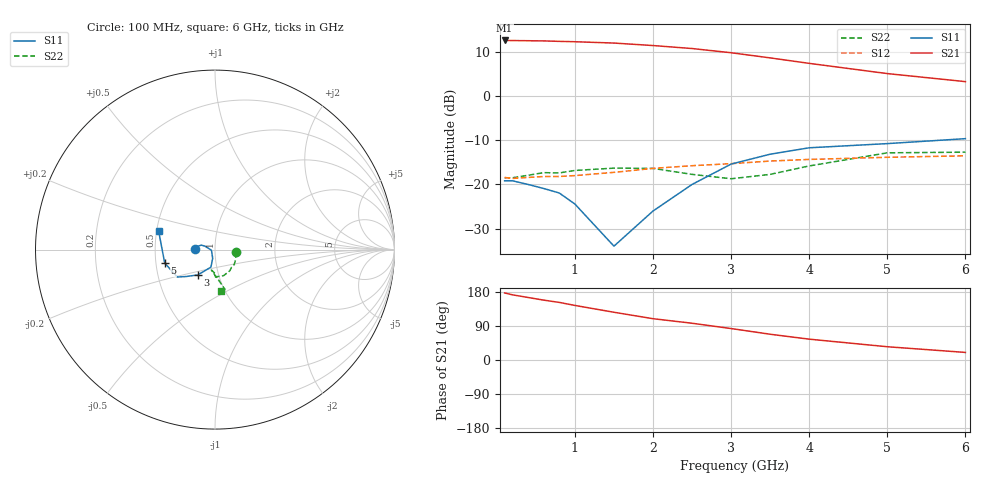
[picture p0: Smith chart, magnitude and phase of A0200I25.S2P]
!  MSA-0200 S AND NOISE PARAMETERS
!  Id=25mA  LAST UPDATED 07-22-92
# ghz s ma r 50
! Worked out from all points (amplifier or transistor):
!   14 points, 100 MHz to 6 GHz, reference 50 ohm
!   highest |S21| = 12.6 dB at 100 MHz (marker M1)
!   |S21| within 3 dB of that: start of sweep to 3.094 GHz
!   unconditionally stable (mu >= 1): start of sweep to end of sweep
!   at 400 MHz: K = 1.20, MAG = 12.8 dB, |S12| = -18.4 dB
!   at 2 GHz: K = 1.14, MAG = 11.7 dB, |S12| = -16.4 dB
!   at 6 GHz: K = 1.47, MAG = 4.3 dB, |S12| = -13.5 dB
!   lowest NFmin = 6.00 dB at 100 MHz
!   S11 on the Smith chart (normalised r, x): 100 MHz: 0.80, +0.00; 3 GHz: 0.80, -0.23; 5 GHz: 0.56, -0.09; 6 GHz: 0.51, +0.12
0.1  0.11 179.0  4.27 177.0  0.12 1.0  0.119 -7.0
0.2  0.11 174.0  4.26 172.0  0.117 4.0  0.119 -12.0
0.4  0.1 170.0  4.24 165.0  0.12 5.0  0.127 -25.0
0.6  0.09 166.0  4.22 158.0  0.123 7.0  0.136 -38.0
0.8  0.08 162.0  4.17 152.0  0.123 10.0  0.135 -47.0
1  0.06 161.0  4.13 144.0  0.126 13.0  0.144 -55.0
1.5  0.02 -170.0  3.99 126.0  0.137 17.0  0.153 -72.0
2  0.05 -105.0  3.74 109.0  0.152 20.0  0.152 -89.0
2.5  0.1 -103.0  3.46 97.0  0.163 25.0  0.13 -91.0
3  0.17 -124.0  3.1 83.0  0.172 26.0  0.116 -100.0
3.5  0.22 -137.0  2.71 68.0  0.184 22.0  0.13 -94.0
4  0.26 -144.0  2.35 55.0  0.192 22.0  0.162 -85.0
5  0.29 -165.0  1.8 35.0  0.203 17.0  0.228 -76.0
6  0.33 162.0  1.46 20.0  0.211 14.0  0.232 -82.0
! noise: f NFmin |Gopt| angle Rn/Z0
0.1  6  0.08  0  1.13
0.5  6.3  0.08  2  1.13
1  6.5  0.07  0  1.12
2  6.9  0.05  -4  1.01
